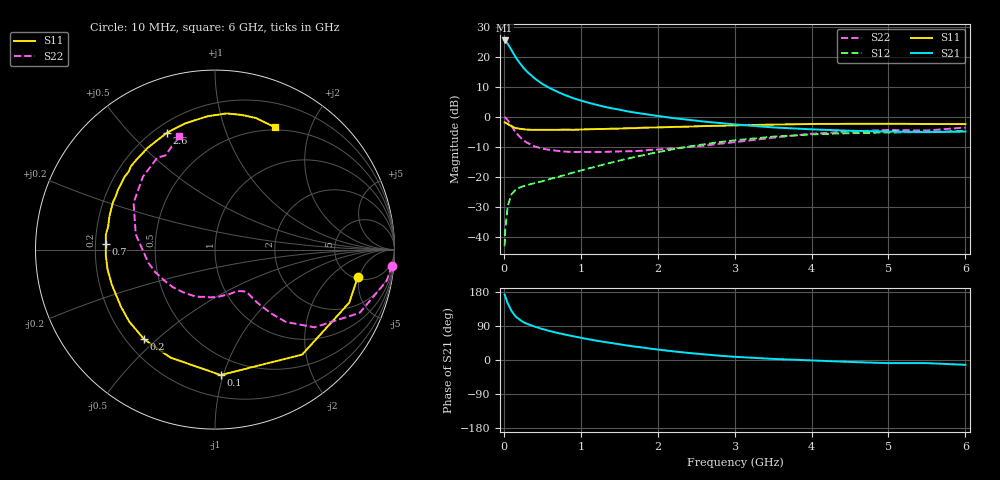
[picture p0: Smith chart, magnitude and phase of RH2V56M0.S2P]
! SIEMENS Small Signal Semiconductors
! BFR106
! Si NPN RF Bipolar Junction Transistor in SOT23
! VCE = 2.5 V  IC = 6 mA
! Common Emitter S-Parameters:  August  1996
# GHz  S  MA  R  50
!  f  S11  S21  S12  S22
! GHz  MAG  ANG  MAG  ANG  MAG  ANG  MAG  ANG
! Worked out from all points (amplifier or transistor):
!   36 points, 10 MHz to 6 GHz, reference 50 ohm
!   highest |S21| = 25.5 dB at 10 MHz (marker M1)
!   |S21| within 3 dB of that: start of sweep to 94.45 MHz
!   unconditionally stable (mu >= 1): 584.9 MHz to 2.141 GHz; 4.515 GHz to end of sweep
!   at 250 MHz: K = 0.56, MSG = 19.8 dB, |S12| = -23.1 dB
!   at 1.4 GHz: K = 1.14, MAG = 6.8 dB, |S12| = -15.2 dB
!   at 6 GHz: K = 1.02, MAG = -1.0 dB, |S12| = -4.7 dB
!   S11 on the Smith chart (normalised r, x): 10 MHz: 5.26, -4.67; 100 MHz: 0.36, -0.98; 200 MHz: 0.27, -0.46; 700 MHz: 0.24, +0.02; 2.6 GHz: 0.25, +0.64; 6 GHz: 0.47, +1.51
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0.01  0.8095 -10.9  18.79 172.7  0.007 86.4  0.99 -5.2
0.02  0.804 -21.6  18.56 167.1  0.0139 79.7  0.9723 -10.3
0.05  0.7604 -50.3  16.56 149.5  0.0322 65.3  0.88 -23.6
0.1  0.6995 -87.4  12.94 129.5  0.0515 51.4  0.7033 -38.0
0.15  0.6508 -112.4  10.05 115.6  0.0604 43.3  0.5638 -45.6
0.2  0.6371 -128.3  8.114 107.3  0.0658 39.9  0.4758 -48.6
0.25  0.6238 -140.1  6.69 100.4  0.0697 38.6  0.4115 -50.4
0.3  0.6133 -148.4  5.7 95.7  0.0728 39.0  0.3727 -51.6
0.4  0.6072 -161.2  4.392 88.2  0.0787 40.8  0.3212 -52.5
0.5  0.6088 -169.7  3.548 81.8  0.0845 43.3  0.2946 -53.5
0.6  0.6092 -177.1  3.004 76.3  0.0923 46.0  0.2814 -55.6
0.7  0.6087 177.1  2.608 71.3  0.0996 48.8  0.2714 -58.5
0.9  0.6091 167.6  2.057 62.7  0.118 52.9  0.2601 -64.3
1.1  0.6212 158.7  1.72 54.9  0.1379 55.9  0.2606 -72.6
1.3  0.6282 151.4  1.483 47.8  0.1612 57.5  0.2602 -81.1
1.6  0.6464 141.5  1.241 38.3  0.2003 58.1  0.2673 -95.8
2.2  0.6796 123.6  0.956 22.9  0.2889 53.6  0.2972 -127.0
2.6  0.7036 112.4  0.836 15.0  0.3491 47.8  0.331 -148.7
3.5  0.7436 93.4  0.668 2.9  0.4685 31.8  0.4499 169.1
4.5  0.7649 78.7  0.587 -5.1  0.5345 13.8  0.571 134.7
5.5  0.7604 67.3  0.557 -8.3  0.5583 2.8  0.5927 117.8
6  0.7589 63.7  0.569 -12.7  0.5836 -4.7  0.6648 107.4
